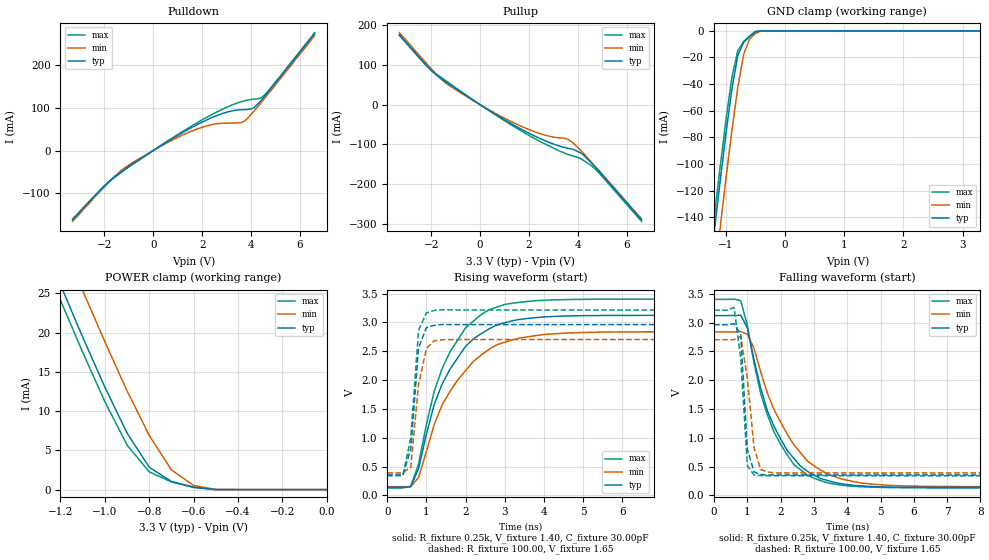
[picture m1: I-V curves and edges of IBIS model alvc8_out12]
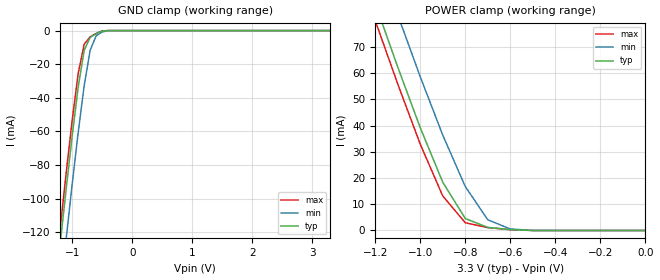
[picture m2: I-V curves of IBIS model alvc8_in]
| IBIS file 62835af.ibs created by s2ibis2 version 1.1
| North Carolina State University Electronics Research Laboratory  1995
[IBIS ver]   2.1
[File name]   74alvcf62835af.ibs
[File Rev]   1.0
[Date]   03/01/99 rtk rtk
[Source]   Integrated Device Technology, Inc.
[Notes]   1.Temperatures: typ=25C, min=100C, max=0C 2.RRmp rates based
   on 50 ohm load.
[Disclaimer] Integrated Device Technology, Inc. ("IDT") hereby grants the
   user of this IBIS model a non-exclusive, nontransferable
   license to use this IBIS model under the following terms. The
   user is granted this license only to use the IBIS model and is
   not granted rights to sell, copy (except as needed to run the
   IBIS model), rent, lease or sub-license the IBIS model in
   whole or in part, or in modified form to anyone. The User may
   modify the IBIS model to suit its specific applications, but
   rights to derivative works and such modifications shall belong
   to IDT. This IBIS model is provided on an AS IS" basis and IDT
   makes absolutely no warranty with respect to the information
   contained herein. IDT DISCLAIMS AND CUSTOMER WAIVES ALL
   WARRANTIES, EXPRESS AND IMPLIED, INCLUDING WARRANTIES OF
   MERCHANTABILITY AND FITNESS FOR A PARTICULAR PURPOSE. THE
   ENTIRE RISK AS TO QUALITY AND PERFORMANCE IS WITH THE USER
   ACCORDINGLY, IN NO EVENT SHALL IDT BE LIABLE FOR ANY DIRECT OR
   INDIRECT DAMAGES, WHETHER IN CONTRACT OR TORT, INCLUDING ANY
   LOST PROFITS OR OTHER INCIDENTAL, CONSEQUENTIAL, EXEMPLARY, OR
   PUNITIVE DAMAGES ARISING OUT OF THE USE OR APPLICATION OF THE
   IBIS model. Further, IDT reserves the right to make changes
   without notice to any product herein to improve reliability,
   function, or design. IDT does not convey any license under
   patent rights or any other intellectual property rights,
   including those of third parties. IDT is not obligated to
   provide maintenance or support for the licensed IBIS model.
[Copyright]   Copyright 1997, Integrated Device Technology, Inc. all rights
   reserved
|   Component ALVCF162835
[Component]   ALVCF162835
[Manufacturer]   Integrated Device Technology
[Package]
| PA56
| variable   typ   min   max
R_pkg   6.50m   5.00m   10.00m
L_pkg   3.30nH   2.50nH   4.90nH
C_pkg   0.29pF   0.010pF   1.16pF
[Pin]  signal_name   model_name   R_pin   L_pin   C_pin
1   NC   nc
2   NC   nc
3   Y1   alvc8_out12
4   GND   GND
5   Y2   alvc8_out12
6   Y3   alvc8_out12
7   VCC   POWER
8   Y4   alvc8_out12
9   Y5   alvc8_out12
10   Y6   alvc8_out12
11   GND   GND
12   Y7   alvc8_out12
13   Y8   alvc8_out12
14   Y9   alvc8_out12
15   Y10   alvc8_out12
16   Y11   alvc8_out12
17   Y12   alvc8_out12
18   GND   GND
19   Y13   alvc8_out12
20   Y14   alvc8_out12
21   Y15   alvc8_out12
22   VCC   POWER
23   Y16   alvc8_out12
24   Y17   alvc8_out12
25   GND   GND
26   Y18   alvc8_out12
27   OEB   alvc8_in
28   LE   alvc8_in
29   GND   GND
30   CLK   alvc8_in
31   A18   alvc8_in
32   GND   GND
33   A17   alvc8_in
34   A16   alvc8_in
35   VCC   POWER
36   A15   alvc8_in
37   A14   alvc8_in
38   A13   alvc8_in
39   GND   GND
40   A12   alvc8_in
41   A11   alvc8_in
42   A10   alvc8_in
43   A9   alvc8_in
44   A8   alvc8_in
45   A7   alvc8_in
46   GND   GND
47   A6   alvc8_in
48   A5   alvc8_in
49   A4   alvc8_in
50   VCC   POWER
51   A3   alvc8_in
52   A2   alvc8_in
53   GND   GND
54   A1   alvc8_in
55   NC   NC
56   GND   GND
| Models and submodels in the file (2): alvc8_out12 (3-state), alvc8_in (Input)
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| in   in   dummy_model
| oe   oe   dummy_model
|   Model alvc8_out12
[Model]   alvc8_out12
Model_type   3-state
Polarity   Non-Inverting
Enable   Active-High
Vmeas =  1.500V
C_comp   3.00pF   NA   NA
[Temperature Range]   25.00   100.00   0.000
[Voltage Range]   3.30V   3.00V   3.60V
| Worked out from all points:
|   slope of the pulldown table from 0 to 0.495 V, typ, clamps not added: 27.6 ohm
|   slope of the pullup table from 0 to 0.495 V, typ, clamps not added: 25.8 ohm
|   GND clamp passes 1 mA (typ) near -0.51 V on its own axis
|   POWER clamp passes 1 mA (typ) near -0.69 V on its own axis
|   rising waveform, R_fixture 0.25k, V_fixture 1.40, C_fixture 30.00pF: 20-80 % time 1.05ns typ, 1.2ns min, 980ps max; typ from 0.138 V to 3.12 V
|   rising waveform, R_fixture 100.00, V_fixture 1.65: 20-80 % time 178ps typ, 250ps min, 201ps max; typ from 0.356 V to 2.96 V
|   falling waveform, R_fixture 0.25k, V_fixture 1.40, C_fixture 30.00pF: 20-80 % time 1.12ns typ, 1.35ns min, 1.05ns max; typ from 3.12 V to 0.138 V
|   falling waveform, R_fixture 100.00, V_fixture 1.65: 20-80 % time 157ps typ, 252ps min, 217ps max; typ from 2.96 V to 0.356 V
[Pulldown]
| voltage   I(typ)   I(min)   I(max)
-3.3V     -161mA     -165mA     -160mA
-1.8V     -71.5mA    -73.3mA    -72.6mA
-1.3V     -49.1mA    -46.1mA    -50.8mA
-600mV    -22.1mA    -19.8mA    -23.1mA
800mV     28.5mA     25mA       30mA
1.9V      63.5mA     52.4mA     68.3mA
3V        89.4mA     63.9mA     101mA
3.7V      95.4mA     67.5mA     115mA
4.1V      99.1mA     90.7mA     120mA
4.4V      116mA      111mA      123mA
4.6V      130mA      125mA      132mA
6.6V      273mA      268mA      275mA
[Pullup]
| voltage   I(typ)   I(min)   I(max)
-3.3V     176mA      181mA      174mA
-1.9V     80.3mA     83.6mA     82mA
-1.5V     61.8mA     58.9mA     64.3mA
-1V       40.8mA     37.7mA     42.5mA
400mV     -15.6mA    -14.2mA    -16.4mA
1.7V      -62.2mA    -54.9mA    -66.6mA
2.9V      -96.6mA    -80.2mA    -106mA
3.5V      -108mA     -85.3mA    -123mA
3.8V      -112mA     -96mA      -129mA
4.2V      -125mA     -121mA     -139mA
4.7V      -156mA     -155mA     -161mA
6.6V      -289mA     -287mA     -293mA
[GND_clamp]
| voltage   I(typ)   I(min)   I(max)
-3.3V     -1.007A    -1.04A     -997mA
-1.3V     -191mA     -226mA     -180mA
-1.2V     -152mA     -187mA     -141mA
-1.1V     -114mA     -149mA     -103mA
-1V       -77.54mA   -111mA     -67.03mA
-900mV    -44.06mA   -75.31mA   -35.25mA
-800mV    -18.73mA   -42.66mA   -14.81mA
-700mV    -8.526mA   -17.61mA   -7.964mA
-600mV    -4.327mA   -6.305mA   -3.891mA
-500mV    -756uA     -1.886mA   -436uA
-400mV    -8.73nA    -25.29uA   -695pA
3.3V      92.41pA    19.42nA    79.2pA
[POWER_clamp]
| voltage   I(typ)   I(min)   I(max)
-3.3V     175mA      181mA      173mA
-1.3V     32.91mA    38.88mA    30.95mA
-1.2V     26.11mA    32.08mA    24.16mA
-1.1V     19.45mA    25.38mA    17.52mA
-1V       13.07mA    18.85mA    11.22mA
-900mV    7.211mA    12.6mA     5.686mA
-800mV    2.858mA    6.904mA    2.259mA
-700mV    1.039mA    2.515mA    986uA
-600mV    306uA      524uA      278uA
-500mV    40.14nA    12.11uA    3.53nA
0V        92.41pA    138pA      101pA
[Ramp]
| variable   typ   min   max
dV/dt_r   1.29/0.24n   1.13/0.30n   1.44/0.25n
dV/dt_f   1.26/0.26n   1.08/0.26n   1.40/0.24n
R_load = 50.00
[Rising Waveform]
R_fixture = 0.25k
V_fixture = 1.40
C_fixture = 30.00pF
R_dut = 7.00m
L_dut = 3.30nH
C_dut = 0.29pF
| time   V(typ)   V(min)   V(max)
0s        138mV      152mV      132mV
600ps     154mV      154mV      155mV
800ps     468mV      312mV      549mV
1.2ns     1.581V     1.23V      1.809V
1.6ns     2.187V     1.801V     2.489V
2ns       2.587V     2.166V     2.908V
2.2ns     2.717V     2.327V     3.025V
3ns       2.995V     2.658V     3.313V
5.4ns     3.121V     2.832V     3.404V
19.8ns    3.124V     2.839V     3.405V
[Rising Waveform]
R_fixture = 100.00
V_fixture = 1.65
R_dut = 7.00m
L_dut = 3.30nH
C_dut = 0.29pF
| time   V(typ)   V(min)   V(max)
0s        356mV      391mV      343mV
400ps     356mV      392mV      344mV
600ps     806mV      494mV      1V
800ps     2.563V     1.932V     2.866V
1ns       2.912V     2.55V      3.166V
1.2ns     2.951V     2.684V     3.21V
1.4ns     2.965V     2.7V       3.222V
1.8ns     2.963V     2.704V     3.218V
19.8ns    2.963V     2.704V     3.218V
[Falling Waveform]
R_fixture = 0.25k
V_fixture = 1.40
C_fixture = 30.00pF
R_dut = 7.00m
L_dut = 3.30nH
C_dut = 0.29pF
| time   V(typ)   V(min)   V(max)
0s        3.124V     2.839V     3.405V
800ps     3.13V      2.846V     3.383V
1ns       2.909V     2.8V       2.955V
1.2ns     2.353V     2.557V     2.296V
1.4ns     1.866V     2.145V     1.771V
1.8ns     1.2V       1.489V     1.106V
2.4ns     642mV      879mV      534mV
3.4ns     261mV      376mV      220mV
5.8ns     142mV      164mV      135mV
19.8ns    138mV      152mV      132mV
[Falling Waveform]
R_fixture = 100.00
V_fixture = 1.65
R_dut = 7.00m
L_dut = 3.30nH
C_dut = 0.29pF
| time   V(typ)   V(min)   V(max)
0s        2.963V     2.704V     3.218V
400ps     2.963V     2.704V     3.218V
600ps     2.983V     2.705V     3.264V
800ps     2.795V     2.761V     2.38V
1ns       801mV      2.038V     518mV
1.2ns     409mV      830mV      356mV
1.4ns     364mV      449mV      345mV
1.6ns     357mV      410mV      343mV
1.8ns     356mV      390mV      343mV
19.8ns    356mV      391mV      343mV
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|   Model alvc8_in
[Model]   alvc8_in
Model_type   Input
Vinl =  0.800V
Vinh =  2.000V
C_comp   3.00pF   NA   NA
[Temperature Range]   25.00   100.00   0.000
[Voltage Range]   3.30V   3.00V   3.60V
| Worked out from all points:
|   GND clamp passes 1 mA (typ) near -0.54 V on its own axis
|   POWER clamp passes 1 mA (typ) near -0.68 V on its own axis
[GND_clamp]
| voltage   I(typ)   I(min)   I(max)
-3.3V     -860mA     -887mA     -851mA
-1.3V     -161mA     -190mA     -151mA
-1.2V     -127mA     -157mA     -118mA
-1.1V     -94.41mA   -124mA     -84.85mA
-1V       -62.78mA   -91.54mA   -53.52mA
-900mV    -33.71mA   -60.78mA   -25.6mA
-800mV    -11.74mA   -32.83mA   -8.09mA
-700mV    -4.033mA   -11.65mA   -3.7mA
-600mV    -1.899mA   -3.108mA   -1.699mA
-500mV    -308uA     -810uA     -172uA
-400mV    -3.848nA   -9.872uA   -399pA
3.3V      39.6pA     19.33nA    26.4pA
[POWER_clamp]
| voltage   I(typ)   I(min)   I(max)
-3.3V     630mA      648mA      624mA
-1.2V     86.56mA    106mA      80.02mA
-1.1V     62.33mA    82.22mA    55.88mA
-1V       39.2mA     58.61mA    32.91mA
-900mV    18.4mA     36.35mA    13.15mA
-800mV    4.556mA    16.76mA    2.954mA
-700mV    1.164mA    4.056mA    1.087mA
-600mV    320uA      578uA      299uA
-500mV    40.08nA    12.23uA    3.465nA
0V        39.6pA     59.11pA    43.2pA
